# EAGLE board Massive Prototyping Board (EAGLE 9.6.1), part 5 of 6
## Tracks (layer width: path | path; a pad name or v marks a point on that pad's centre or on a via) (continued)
N$1626  (via drill 0.94)
  Bottom 2.032: v262.89,220.98 v265.43,220.98 v267.97,220.98 v270.51,220.98 v273.05,220.98
N$1627  (via drill 0.94)
  Bottom 2.032: v262.89,223.52 v265.43,223.52 v267.97,223.52 v270.51,223.52 v273.05,223.52
N$1628  (via drill 0.94)
  Bottom 2.032: v262.89,226.06 v265.43,226.06 v267.97,226.06 v270.51,226.06 v273.05,226.06
N$1629  (via drill 0.94)
  Bottom 2.032: v262.89,228.6 v265.43,228.6 v267.97,228.6 v270.51,228.6 v273.05,228.6
N$1630  (via drill 0.94)
  Bottom 2.032: v262.89,231.14 v265.43,231.14 v267.97,231.14 v270.51,231.14 v273.05,231.14
N$1631  (via drill 0.94)
  Bottom 2.032: v262.89,233.68 v265.43,233.68 v267.97,233.68 v270.51,233.68 v273.05,233.68
N$1632  (via drill 0.94)
  Bottom 2.032: v262.89,236.22 v265.43,236.22 v267.97,236.22 v270.51,236.22 v273.05,236.22
N$1633  (via drill 0.94)
  Bottom 2.032: v262.89,238.76 v265.43,238.76 v267.97,238.76 v270.51,238.76 v273.05,238.76
N$1634  (via drill 0.94)
  Bottom 2.032: v262.89,241.3 v265.43,241.3 v267.97,241.3 v270.51,241.3 v273.05,241.3
N$1635  (via drill 0.94)
  Bottom 2.032: v262.89,243.84 v265.43,243.84 v267.97,243.84 v270.51,243.84 v273.05,243.84
N$1636  (via drill 0.94)
  Bottom 2.032: v262.89,246.38 v265.43,246.38 v267.97,246.38 v270.51,246.38 v273.05,246.38
N$1637  (via drill 0.94)
  Bottom 2.032: v262.89,248.92 v265.43,248.92 v267.97,248.92 v270.51,248.92 v273.05,248.92
N$1638  (via drill 0.94)
  Bottom 2.032: v262.89,251.46 v265.43,251.46 v267.97,251.46 v270.51,251.46 v273.05,251.46
N$1639  (via drill 0.94)
  Bottom 2.032: v262.89,254 v265.43,254 v267.97,254 v270.51,254 v273.05,254
N$1640  (via drill 0.94)
  Bottom 2.032: v262.89,256.54 v265.43,256.54 v267.97,256.54 v270.51,256.54 v273.05,256.54
N$1641  (via drill 0.94)
  Bottom 2.032: v262.89,259.08 v265.43,259.08 v267.97,259.08 v270.51,259.08 v273.05,259.08
N$1642  (via drill 0.94)
  Bottom 2.032: v262.89,261.62 v265.43,261.62 v267.97,261.62 v270.51,261.62 v273.05,261.62
N$1643  (via drill 0.94)
  Bottom 2.032: v262.89,264.16 v265.43,264.16 v267.97,264.16 v270.51,264.16 v273.05,264.16
N$1644  (via drill 0.94)
  Bottom 2.032: v262.89,266.7 v265.43,266.7 v267.97,266.7 v270.51,266.7 v273.05,266.7
N$1645  (via drill 0.94)
  Bottom 2.032: v262.89,269.24 v265.43,269.24 v267.97,269.24 v270.51,269.24 v273.05,269.24
N$1646  (via drill 0.94)
  Bottom 2.032: v262.89,271.78 v265.43,271.78 v267.97,271.78 v270.51,271.78 v273.05,271.78
N$1647  (via drill 0.94)
  Bottom 2.032: v262.89,274.32 v265.43,274.32 v267.97,274.32 v270.51,274.32 v273.05,274.32
N$1648  (via drill 0.94)
  Bottom 2.032: v262.89,276.86 v265.43,276.86 v267.97,276.86 v270.51,276.86 v273.05,276.86
N$1649  (via drill 0.94)
  Bottom 2.032: v280.67,12.7 v283.21,12.7 v285.75,12.7 v288.29,12.7 v290.83,12.7
N$1650  (via drill 0.94)
  Bottom 2.032: v280.67,15.24 v283.21,15.24 v285.75,15.24 v288.29,15.24 v290.83,15.24
N$1651  (via drill 0.94)
  Bottom 2.032: v280.67,17.78 v283.21,17.78 v285.75,17.78 v288.29,17.78 v290.83,17.78
N$1652  (via drill 0.94)
  Bottom 2.032: v280.67,20.32 v283.21,20.32 v285.75,20.32 v288.29,20.32 v290.83,20.32
N$1653  (via drill 0.94)
  Bottom 2.032: v280.67,22.86 v283.21,22.86 v285.75,22.86 v288.29,22.86 v290.83,22.86
N$1654  (via drill 0.94)
  Bottom 2.032: v280.67,25.4 v283.21,25.4 v285.75,25.4 v288.29,25.4 v290.83,25.4
N$1655  (via drill 0.94)
  Bottom 2.032: v280.67,27.94 v283.21,27.94 v285.75,27.94 v288.29,27.94 v290.83,27.94
N$1656  (via drill 0.94)
  Bottom 2.032: v280.67,30.48 v283.21,30.48 v285.75,30.48 v288.29,30.48 v290.83,30.48
N$1657  (via drill 0.94)
  Bottom 2.032: v280.67,33.02 v283.21,33.02 v285.75,33.02 v288.29,33.02 v290.83,33.02
N$1658  (via drill 0.94)
  Bottom 2.032: v280.67,35.56 v283.21,35.56 v285.75,35.56 v288.29,35.56 v290.83,35.56
N$1659  (via drill 0.94)
  Bottom 2.032: v280.67,38.1 v283.21,38.1 v285.75,38.1 v288.29,38.1 v290.83,38.1
N$1660  (via drill 0.94)
  Bottom 2.032: v280.67,40.64 v283.21,40.64 v285.75,40.64 v288.29,40.64 v290.83,40.64
N$1661  (via drill 0.94)
  Bottom 2.032: v280.67,43.18 v283.21,43.18 v285.75,43.18 v288.29,43.18 v290.83,43.18
N$1662  (via drill 0.94)
  Bottom 2.032: v280.67,45.72 v283.21,45.72 v285.75,45.72 v288.29,45.72 v290.83,45.72
N$1663  (via drill 0.94)
  Bottom 2.032: v280.67,48.26 v283.21,48.26 v285.75,48.26 v288.29,48.26 v290.83,48.26
N$1664  (via drill 0.94)
  Bottom 2.032: v280.67,50.8 v283.21,50.8 v285.75,50.8 v288.29,50.8 v290.83,50.8
N$1665  (via drill 0.94)
  Bottom 2.032: v280.67,53.34 v283.21,53.34 v285.75,53.34 v288.29,53.34 v290.83,53.34
N$1666  (via drill 0.94)
  Bottom 2.032: v280.67,55.88 v283.21,55.88 v285.75,55.88 v288.29,55.88 v290.83,55.88
N$1667  (via drill 0.94)
  Bottom 2.032: v280.67,58.42 v283.21,58.42 v285.75,58.42 v288.29,58.42 v290.83,58.42
N$1668  (via drill 0.94)
  Bottom 2.032: v280.67,60.96 v283.21,60.96 v285.75,60.96 v288.29,60.96 v290.83,60.96
N$1669  (via drill 0.94)
  Bottom 2.032: v280.67,63.5 v283.21,63.5 v285.75,63.5 v288.29,63.5 v290.83,63.5
N$1670  (via drill 0.94)
  Bottom 2.032: v280.67,66.04 v283.21,66.04 v285.75,66.04 v288.29,66.04 v290.83,66.04
N$1671  (via drill 0.94)
  Bottom 2.032: v280.67,68.58 v283.21,68.58 v285.75,68.58 v288.29,68.58 v290.83,68.58
N$1672  (via drill 0.94)
  Bottom 2.032: v280.67,71.12 v283.21,71.12 v285.75,71.12 v288.29,71.12 v290.83,71.12
N$1673  (via drill 0.94)
  Bottom 2.032: v280.67,73.66 v283.21,73.66 v285.75,73.66 v288.29,73.66 v290.83,73.66
N$1674  (via drill 0.94)
  Bottom 2.032: v280.67,76.2 v283.21,76.2 v285.75,76.2 v288.29,76.2 v290.83,76.2
N$1675  (via drill 0.94)
  Bottom 2.032: v280.67,78.74 v283.21,78.74 v285.75,78.74 v288.29,78.74 v290.83,78.74
N$1676  (via drill 0.94)
  Bottom 2.032: v280.67,81.28 v283.21,81.28 v285.75,81.28 v288.29,81.28 v290.83,81.28
N$1677  (via drill 0.94)
  Bottom 2.032: v280.67,83.82 v283.21,83.82 v285.75,83.82 v288.29,83.82 v290.83,83.82
N$1678  (via drill 0.94)
  Bottom 2.032: v280.67,86.36 v283.21,86.36 v285.75,86.36 v288.29,86.36 v290.83,86.36
N$1679  (via drill 0.94)
  Bottom 2.032: v280.67,88.9 v283.21,88.9 v285.75,88.9 v288.29,88.9 v290.83,88.9
N$1680  (via drill 0.94)
  Bottom 2.032: v280.67,91.44 v283.21,91.44 v285.75,91.44 v288.29,91.44 v290.83,91.44
N$1681  (via drill 0.94)
  Bottom 2.032: v280.67,93.98 v283.21,93.98 v285.75,93.98 v288.29,93.98 v290.83,93.98
N$1682  (via drill 0.94)
  Bottom 2.032: v280.67,96.52 v283.21,96.52 v285.75,96.52 v288.29,96.52 v290.83,96.52
N$1683  (via drill 0.94)
  Bottom 2.032: v280.67,99.06 v283.21,99.06 v285.75,99.06 v288.29,99.06 v290.83,99.06
N$1684  (via drill 0.94)
  Bottom 2.032: v280.67,101.6 v283.21,101.6 v285.75,101.6 v288.29,101.6 v290.83,101.6
N$1685  (via drill 0.94)
  Bottom 2.032: v280.67,104.14 v283.21,104.14 v285.75,104.14 v288.29,104.14 v290.83,104.14
N$1686  (via drill 0.94)
  Bottom 2.032: v280.67,106.68 v283.21,106.68 v285.75,106.68 v288.29,106.68 v290.83,106.68
N$1687  (via drill 0.94)
  Bottom 2.032: v280.67,109.22 v283.21,109.22 v285.75,109.22 v288.29,109.22 v290.83,109.22
N$1688  (via drill 0.94)
  Bottom 2.032: v280.67,111.76 v283.21,111.76 v285.75,111.76 v288.29,111.76 v290.83,111.76
N$1689  (via drill 0.94)
  Bottom 2.032: v280.67,114.3 v283.21,114.3 v285.75,114.3 v288.29,114.3 v290.83,114.3
N$1690  (via drill 0.94)
  Bottom 2.032: v280.67,116.84 v283.21,116.84 v285.75,116.84 v288.29,116.84 v290.83,116.84
N$1691  (via drill 0.94)
  Bottom 2.032: v280.67,119.38 v283.21,119.38 v285.75,119.38 v288.29,119.38 v290.83,119.38
N$1692  (via drill 0.94)
  Bottom 2.032: v280.67,121.92 v283.21,121.92 v285.75,121.92 v288.29,121.92 v290.83,121.92
N$1693  (via drill 0.94)
  Bottom 2.032: v280.67,124.46 v283.21,124.46 v285.75,124.46 v288.29,124.46 v290.83,124.46
N$1694  (via drill 0.94)
  Bottom 2.032: v280.67,127 v283.21,127 v285.75,127 v288.29,127 v290.83,127
N$1695  (via drill 0.94)
  Bottom 2.032: v280.67,129.54 v283.21,129.54 v285.75,129.54 v288.29,129.54 v290.83,129.54
N$1696  (via drill 0.94)
  Bottom 2.032: v280.67,132.08 v283.21,132.08 v285.75,132.08 v288.29,132.08 v290.83,132.08
N$1697  (via drill 0.94)
  Bottom 2.032: v280.67,134.62 v283.21,134.62 v285.75,134.62 v288.29,134.62 v290.83,134.62
N$1698  (via drill 0.94)
  Bottom 2.032: v280.67,137.16 v283.21,137.16 v285.75,137.16 v288.29,137.16 v290.83,137.16
N$1699  (via drill 0.94)
  Bottom 2.032: v280.67,139.7 v283.21,139.7 v285.75,139.7 v288.29,139.7 v290.83,139.7
N$1700  (via drill 0.94)
  Bottom 2.032: v280.67,142.24 v283.21,142.24 v285.75,142.24 v288.29,142.24 v290.83,142.24
N$1701  (via drill 0.94)
  Bottom 2.032: v280.67,144.78 v283.21,144.78 v285.75,144.78 v288.29,144.78 v290.83,144.78
N$1702  (via drill 0.94)
  Bottom 2.032: v280.67,147.32 v283.21,147.32 v285.75,147.32 v288.29,147.32 v290.83,147.32
N$1703  (via drill 0.94)
  Bottom 2.032: v280.67,149.86 v283.21,149.86 v285.75,149.86 v288.29,149.86 v290.83,149.86
N$1704  (via drill 0.94)
  Bottom 2.032: v280.67,152.4 v283.21,152.4 v285.75,152.4 v288.29,152.4 v290.83,152.4
N$1705  (via drill 0.94)
  Bottom 2.032: v280.67,154.94 v283.21,154.94 v285.75,154.94 v288.29,154.94 v290.83,154.94
N$1706  (via drill 0.94)
  Bottom 2.032: v280.67,157.48 v283.21,157.48 v285.75,157.48 v288.29,157.48 v290.83,157.48
N$1707  (via drill 0.94)
  Bottom 2.032: v280.67,160.02 v283.21,160.02 v285.75,160.02 v288.29,160.02 v290.83,160.02
N$1708  (via drill 0.94)
  Bottom 2.032: v280.67,162.56 v283.21,162.56 v285.75,162.56 v288.29,162.56 v290.83,162.56
N$1709  (via drill 0.94)
  Bottom 2.032: v280.67,165.1 v283.21,165.1 v285.75,165.1 v288.29,165.1 v290.83,165.1
N$1710  (via drill 0.94)
  Bottom 2.032: v280.67,167.64 v283.21,167.64 v285.75,167.64 v288.29,167.64 v290.83,167.64
N$1711  (via drill 0.94)
  Bottom 2.032: v280.67,170.18 v283.21,170.18 v285.75,170.18 v288.29,170.18 v290.83,170.18
N$1712  (via drill 0.94)
  Bottom 2.032: v280.67,172.72 v283.21,172.72 v285.75,172.72 v288.29,172.72 v290.83,172.72
N$1713  (via drill 0.94)
  Bottom 2.032: v280.67,175.26 v283.21,175.26 v285.75,175.26 v288.29,175.26 v290.83,175.26
N$1714  (via drill 0.94)
  Bottom 2.032: v280.67,177.8 v283.21,177.8 v285.75,177.8 v288.29,177.8 v290.83,177.8
N$1715  (via drill 0.94)
  Bottom 2.032: v280.67,180.34 v283.21,180.34 v285.75,180.34 v288.29,180.34 v290.83,180.34
N$1716  (via drill 0.94)
  Bottom 2.032: v280.67,182.88 v283.21,182.88 v285.75,182.88 v288.29,182.88 v290.83,182.88
N$1717  (via drill 0.94)
  Bottom 2.032: v280.67,185.42 v283.21,185.42 v285.75,185.42 v288.29,185.42 v290.83,185.42
N$1718  (via drill 0.94)
  Bottom 2.032: v280.67,187.96 v283.21,187.96 v285.75,187.96 v288.29,187.96 v290.83,187.96
N$1719  (via drill 0.94)
  Bottom 2.032: v280.67,190.5 v283.21,190.5 v285.75,190.5 v288.29,190.5 v290.83,190.5
N$1720  (via drill 0.94)
  Bottom 2.032: v280.67,193.04 v283.21,193.04 v285.75,193.04 v288.29,193.04 v290.83,193.04
N$1721  (via drill 0.94)
  Bottom 2.032: v280.67,195.58 v283.21,195.58 v285.75,195.58 v288.29,195.58 v290.83,195.58
N$1722  (via drill 0.94)
  Bottom 2.032: v280.67,198.12 v283.21,198.12 v285.75,198.12 v288.29,198.12 v290.83,198.12
N$1723  (via drill 0.94)
  Bottom 2.032: v280.67,200.66 v283.21,200.66 v285.75,200.66 v288.29,200.66 v290.83,200.66
N$1724  (via drill 0.94)
  Bottom 2.032: v280.67,203.2 v283.21,203.2 v285.75,203.2 v288.29,203.2 v290.83,203.2
N$1725  (via drill 0.94)
  Bottom 2.032: v280.67,205.74 v283.21,205.74 v285.75,205.74 v288.29,205.74 v290.83,205.74
N$1726  (via drill 0.94)
  Bottom 2.032: v280.67,208.28 v283.21,208.28 v285.75,208.28 v288.29,208.28 v290.83,208.28
N$1727  (via drill 0.94)
  Bottom 2.032: v280.67,210.82 v283.21,210.82 v285.75,210.82 v288.29,210.82 v290.83,210.82
N$1728  (via drill 0.94)
  Bottom 2.032: v280.67,213.36 v283.21,213.36 v285.75,213.36 v288.29,213.36 v290.83,213.36
N$1729  (via drill 0.94)
  Bottom 2.032: v280.67,215.9 v283.21,215.9 v285.75,215.9 v288.29,215.9 v290.83,215.9
N$1730  (via drill 0.94)
  Bottom 2.032: v280.67,218.44 v283.21,218.44 v285.75,218.44 v288.29,218.44 v290.83,218.44
N$1731  (via drill 0.94)
  Bottom 2.032: v280.67,220.98 v283.21,220.98 v285.75,220.98 v288.29,220.98 v290.83,220.98
N$1732  (via drill 0.94)
  Bottom 2.032: v280.67,223.52 v283.21,223.52 v285.75,223.52 v288.29,223.52 v290.83,223.52
N$1733  (via drill 0.94)
  Bottom 2.032: v280.67,226.06 v283.21,226.06 v285.75,226.06 v288.29,226.06 v290.83,226.06
N$1734  (via drill 0.94)
  Bottom 2.032: v280.67,228.6 v283.21,228.6 v285.75,228.6 v288.29,228.6 v290.83,228.6
N$1735  (via drill 0.94)
  Bottom 2.032: v280.67,231.14 v283.21,231.14 v285.75,231.14 v288.29,231.14 v290.83,231.14
N$1736  (via drill 0.94)
  Bottom 2.032: v280.67,233.68 v283.21,233.68 v285.75,233.68 v288.29,233.68 v290.83,233.68
N$1737  (via drill 0.94)
  Bottom 2.032: v280.67,236.22 v283.21,236.22 v285.75,236.22 v288.29,236.22 v290.83,236.22
N$1738  (via drill 0.94)
  Bottom 2.032: v280.67,238.76 v283.21,238.76 v285.75,238.76 v288.29,238.76 v290.83,238.76
N$1739  (via drill 0.94)
  Bottom 2.032: v280.67,241.3 v283.21,241.3 v285.75,241.3 v288.29,241.3 v290.83,241.3
N$1740  (via drill 0.94)
  Bottom 2.032: v280.67,243.84 v283.21,243.84 v285.75,243.84 v288.29,243.84 v290.83,243.84
N$1741  (via drill 0.94)
  Bottom 2.032: v280.67,246.38 v283.21,246.38 v285.75,246.38 v288.29,246.38 v290.83,246.38
N$1742  (via drill 0.94)
  Bottom 2.032: v280.67,248.92 v283.21,248.92 v285.75,248.92 v288.29,248.92 v290.83,248.92
N$1743  (via drill 0.94)
  Bottom 2.032: v280.67,251.46 v283.21,251.46 v285.75,251.46 v288.29,251.46 v290.83,251.46
N$1744  (via drill 0.94)
  Bottom 2.032: v280.67,254 v283.21,254 v285.75,254 v288.29,254 v290.83,254
N$1745  (via drill 0.94)
  Bottom 2.032: v280.67,256.54 v283.21,256.54 v285.75,256.54 v288.29,256.54 v290.83,256.54
N$1746  (via drill 0.94)
  Bottom 2.032: v280.67,259.08 v283.21,259.08 v285.75,259.08 v288.29,259.08 v290.83,259.08
N$1747  (via drill 0.94)
  Bottom 2.032: v280.67,261.62 v283.21,261.62 v285.75,261.62 v288.29,261.62 v290.83,261.62
N$1748  (via drill 0.94)
  Bottom 2.032: v280.67,264.16 v283.21,264.16 v285.75,264.16 v288.29,264.16 v290.83,264.16
N$1749  (via drill 0.94)
  Bottom 2.032: v280.67,266.7 v283.21,266.7 v285.75,266.7 v288.29,266.7 v290.83,266.7
N$1750  (via drill 0.94)
  Bottom 2.032: v280.67,269.24 v283.21,269.24 v285.75,269.24 v288.29,269.24 v290.83,269.24
N$1751  (via drill 0.94)
  Bottom 2.032: v280.67,271.78 v283.21,271.78 v285.75,271.78 v288.29,271.78 v290.83,271.78
N$1752  (via drill 0.94)
  Bottom 2.032: v280.67,274.32 v283.21,274.32 v285.75,274.32 v288.29,274.32 v290.83,274.32
N$1753  (via drill 0.94)
  Bottom 2.032: v280.67,276.86 v283.21,276.86 v285.75,276.86 v288.29,276.86 v290.83,276.86
N$1754  (via drill 0.94)
  Bottom 2.032: v293.37,12.7 v295.91,12.7 v298.45,12.7 v300.99,12.7 v303.53,12.7
N$1755  (via drill 0.94)
  Bottom 2.032: v293.37,15.24 v295.91,15.24 v298.45,15.24 v300.99,15.24 v303.53,15.24
N$1756  (via drill 0.94)
  Bottom 2.032: v293.37,17.78 v295.91,17.78 v298.45,17.78 v300.99,17.78 v303.53,17.78
N$1757  (via drill 0.94)
  Bottom 2.032: v293.37,20.32 v295.91,20.32 v298.45,20.32 v300.99,20.32 v303.53,20.32
N$1758  (via drill 0.94)
  Bottom 2.032: v293.37,22.86 v295.91,22.86 v298.45,22.86 v300.99,22.86 v303.53,22.86
N$1759  (via drill 0.94)
  Bottom 2.032: v293.37,25.4 v295.91,25.4 v298.45,25.4 v300.99,25.4 v303.53,25.4
N$1760  (via drill 0.94)
  Bottom 2.032: v293.37,27.94 v295.91,27.94 v298.45,27.94 v300.99,27.94 v303.53,27.94
N$1761  (via drill 0.94)
  Bottom 2.032: v293.37,30.48 v295.91,30.48 v298.45,30.48 v300.99,30.48 v303.53,30.48
N$1762  (via drill 0.94)
  Bottom 2.032: v293.37,33.02 v295.91,33.02 v298.45,33.02 v300.99,33.02 v303.53,33.02
N$1763  (via drill 0.94)
  Bottom 2.032: v293.37,35.56 v295.91,35.56 v298.45,35.56 v300.99,35.56 v303.53,35.56
N$1764  (via drill 0.94)
  Bottom 2.032: v293.37,38.1 v295.91,38.1 v298.45,38.1 v300.99,38.1 v303.53,38.1
N$1765  (via drill 0.94)
  Bottom 2.032: v293.37,40.64 v295.91,40.64 v298.45,40.64 v300.99,40.64 v303.53,40.64
N$1766  (via drill 0.94)
  Bottom 2.032: v293.37,43.18 v295.91,43.18 v298.45,43.18 v300.99,43.18 v303.53,43.18
N$1767  (via drill 0.94)
  Bottom 2.032: v293.37,45.72 v295.91,45.72 v298.45,45.72 v300.99,45.72 v303.53,45.72
N$1768  (via drill 0.94)
  Bottom 2.032: v293.37,48.26 v295.91,48.26 v298.45,48.26 v300.99,48.26 v303.53,48.26
N$1769  (via drill 0.94)
  Bottom 2.032: v293.37,50.8 v295.91,50.8 v298.45,50.8 v300.99,50.8 v303.53,50.8
N$1770  (via drill 0.94)
  Bottom 2.032: v293.37,53.34 v295.91,53.34 v298.45,53.34 v300.99,53.34 v303.53,53.34
N$1771  (via drill 0.94)
  Bottom 2.032: v293.37,55.88 v295.91,55.88 v298.45,55.88 v300.99,55.88 v303.53,55.88
N$1772  (via drill 0.94)
  Bottom 2.032: v293.37,58.42 v295.91,58.42 v298.45,58.42 v300.99,58.42 v303.53,58.42
N$1773  (via drill 0.94)
  Bottom 2.032: v293.37,60.96 v295.91,60.96 v298.45,60.96 v300.99,60.96 v303.53,60.96
N$1774  (via drill 0.94)
  Bottom 2.032: v293.37,63.5 v295.91,63.5 v298.45,63.5 v300.99,63.5 v303.53,63.5
N$1775  (via drill 0.94)
  Bottom 2.032: v293.37,66.04 v295.91,66.04 v298.45,66.04 v300.99,66.04 v303.53,66.04
N$1776  (via drill 0.94)
  Bottom 2.032: v293.37,68.58 v295.91,68.58 v298.45,68.58 v300.99,68.58 v303.53,68.58
N$1777  (via drill 0.94)
  Bottom 2.032: v293.37,71.12 v295.91,71.12 v298.45,71.12 v300.99,71.12 v303.53,71.12
N$1778  (via drill 0.94)
  Bottom 2.032: v293.37,73.66 v295.91,73.66 v298.45,73.66 v300.99,73.66 v303.53,73.66
N$1779  (via drill 0.94)
  Bottom 2.032: v293.37,76.2 v295.91,76.2 v298.45,76.2 v300.99,76.2 v303.53,76.2
N$1780  (via drill 0.94)
  Bottom 2.032: v293.37,78.74 v295.91,78.74 v298.45,78.74 v300.99,78.74 v303.53,78.74
N$1781  (via drill 0.94)
  Bottom 2.032: v293.37,81.28 v295.91,81.28 v298.45,81.28 v300.99,81.28 v303.53,81.28
N$1782  (via drill 0.94)
  Bottom 2.032: v293.37,83.82 v295.91,83.82 v298.45,83.82 v300.99,83.82 v303.53,83.82
N$1783  (via drill 0.94)
  Bottom 2.032: v293.37,86.36 v295.91,86.36 v298.45,86.36 v300.99,86.36 v303.53,86.36
N$1784  (via drill 0.94)
  Bottom 2.032: v293.37,88.9 v295.91,88.9 v298.45,88.9 v300.99,88.9 v303.53,88.9
N$1785  (via drill 0.94)
  Bottom 2.032: v293.37,91.44 v295.91,91.44 v298.45,91.44 v300.99,91.44 v303.53,91.44
N$1786  (via drill 0.94)
  Bottom 2.032: v293.37,93.98 v295.91,93.98 v298.45,93.98 v300.99,93.98 v303.53,93.98
N$1787  (via drill 0.94)
  Bottom 2.032: v293.37,96.52 v295.91,96.52 v298.45,96.52 v300.99,96.52 v303.53,96.52
N$1788  (via drill 0.94)
  Bottom 2.032: v293.37,99.06 v295.91,99.06 v298.45,99.06 v300.99,99.06 v303.53,99.06
N$1789  (via drill 0.94)
  Bottom 2.032: v293.37,101.6 v295.91,101.6 v298.45,101.6 v300.99,101.6 v303.53,101.6
N$1790  (via drill 0.94)
  Bottom 2.032: v293.37,104.14 v295.91,104.14 v298.45,104.14 v300.99,104.14 v303.53,104.14
N$1791  (via drill 0.94)
  Bottom 2.032: v293.37,106.68 v295.91,106.68 v298.45,106.68 v300.99,106.68 v303.53,106.68
N$1792  (via drill 0.94)
  Bottom 2.032: v293.37,109.22 v295.91,109.22 v298.45,109.22 v300.99,109.22 v303.53,109.22
N$1793  (via drill 0.94)
  Bottom 2.032: v293.37,111.76 v295.91,111.76 v298.45,111.76 v300.99,111.76 v303.53,111.76
N$1794  (via drill 0.94)
  Bottom 2.032: v293.37,114.3 v295.91,114.3 v298.45,114.3 v300.99,114.3 v303.53,114.3
N$1795  (via drill 0.94)
  Bottom 2.032: v293.37,116.84 v295.91,116.84 v298.45,116.84 v300.99,116.84 v303.53,116.84
N$1796  (via drill 0.94)
  Bottom 2.032: v293.37,119.38 v295.91,119.38 v298.45,119.38 v300.99,119.38 v303.53,119.38
N$1797  (via drill 0.94)
  Bottom 2.032: v293.37,121.92 v295.91,121.92 v298.45,121.92 v300.99,121.92 v303.53,121.92
N$1798  (via drill 0.94)
  Bottom 2.032: v293.37,124.46 v295.91,124.46 v298.45,124.46 v300.99,124.46 v303.53,124.46
N$1799  (via drill 0.94)
  Bottom 2.032: v293.37,127 v295.91,127 v298.45,127 v300.99,127 v303.53,127
N$1800  (via drill 0.94)
  Bottom 2.032: v293.37,129.54 v295.91,129.54 v298.45,129.54 v300.99,129.54 v303.53,129.54
N$1801  (via drill 0.94)
  Bottom 2.032: v293.37,132.08 v295.91,132.08 v298.45,132.08 v300.99,132.08 v303.53,132.08
N$1802  (via drill 0.94)
  Bottom 2.032: v293.37,134.62 v295.91,134.62 v298.45,134.62 v300.99,134.62 v303.53,134.62
N$1803  (via drill 0.94)
  Bottom 2.032: v293.37,137.16 v295.91,137.16 v298.45,137.16 v300.99,137.16 v303.53,137.16
N$1804  (via drill 0.94)
  Bottom 2.032: v293.37,139.7 v295.91,139.7 v298.45,139.7 v300.99,139.7 v303.53,139.7
N$1805  (via drill 0.94)
  Bottom 2.032: v293.37,142.24 v295.91,142.24 v298.45,142.24 v300.99,142.24 v303.53,142.24
N$1806  (via drill 0.94)
  Bottom 2.032: v293.37,144.78 v295.91,144.78 v298.45,144.78 v300.99,144.78 v303.53,144.78
N$1807  (via drill 0.94)
  Bottom 2.032: v293.37,147.32 v295.91,147.32 v298.45,147.32 v300.99,147.32 v303.53,147.32
N$1808  (via drill 0.94)
  Bottom 2.032: v293.37,149.86 v295.91,149.86 v298.45,149.86 v300.99,149.86 v303.53,149.86
N$1809  (via drill 0.94)
  Bottom 2.032: v293.37,152.4 v295.91,152.4 v298.45,152.4 v300.99,152.4 v303.53,152.4
N$1810  (via drill 0.94)
  Bottom 2.032: v293.37,154.94 v295.91,154.94 v298.45,154.94 v300.99,154.94 v303.53,154.94
N$1811  (via drill 0.94)
  Bottom 2.032: v293.37,157.48 v295.91,157.48 v298.45,157.48 v300.99,157.48 v303.53,157.48
N$1812  (via drill 0.94)
  Bottom 2.032: v293.37,160.02 v295.91,160.02 v298.45,160.02 v300.99,160.02 v303.53,160.02
N$1813  (via drill 0.94)
  Bottom 2.032: v293.37,162.56 v295.91,162.56 v298.45,162.56 v300.99,162.56 v303.53,162.56
N$1814  (via drill 0.94)
  Bottom 2.032: v293.37,165.1 v295.91,165.1 v298.45,165.1 v300.99,165.1 v303.53,165.1
N$1815  (via drill 0.94)
  Bottom 2.032: v293.37,167.64 v295.91,167.64 v298.45,167.64 v300.99,167.64 v303.53,167.64
N$1816  (via drill 0.94)
  Bottom 2.032: v293.37,170.18 v295.91,170.18 v298.45,170.18 v300.99,170.18 v303.53,170.18
N$1817  (via drill 0.94)
  Bottom 2.032: v293.37,172.72 v295.91,172.72 v298.45,172.72 v300.99,172.72 v303.53,172.72
N$1818  (via drill 0.94)
  Bottom 2.032: v293.37,175.26 v295.91,175.26 v298.45,175.26 v300.99,175.26 v303.53,175.26
N$1819  (via drill 0.94)
  Bottom 2.032: v293.37,177.8 v295.91,177.8 v298.45,177.8 v300.99,177.8 v303.53,177.8
N$1820  (via drill 0.94)
  Bottom 2.032: v293.37,180.34 v295.91,180.34 v298.45,180.34 v300.99,180.34 v303.53,180.34
N$1821  (via drill 0.94)
  Bottom 2.032: v293.37,182.88 v295.91,182.88 v298.45,182.88 v300.99,182.88 v303.53,182.88
N$1822  (via drill 0.94)
  Bottom 2.032: v293.37,185.42 v295.91,185.42 v298.45,185.42 v300.99,185.42 v303.53,185.42
N$1823  (via drill 0.94)
  Bottom 2.032: v293.37,187.96 v295.91,187.96 v298.45,187.96 v300.99,187.96 v303.53,187.96
N$1824  (via drill 0.94)
  Bottom 2.032: v293.37,190.5 v295.91,190.5 v298.45,190.5 v300.99,190.5 v303.53,190.5
N$1825  (via drill 0.94)
  Bottom 2.032: v293.37,193.04 v295.91,193.04 v298.45,193.04 v300.99,193.04 v303.53,193.04
N$1826  (via drill 0.94)
  Bottom 2.032: v293.37,195.58 v295.91,195.58 v298.45,195.58 v300.99,195.58 v303.53,195.58
N$1827  (via drill 0.94)
  Bottom 2.032: v293.37,198.12 v295.91,198.12 v298.45,198.12 v300.99,198.12 v303.53,198.12
N$1828  (via drill 0.94)
  Bottom 2.032: v293.37,200.66 v295.91,200.66 v298.45,200.66 v300.99,200.66 v303.53,200.66
N$1829  (via drill 0.94)
  Bottom 2.032: v293.37,203.2 v295.91,203.2 v298.45,203.2 v300.99,203.2 v303.53,203.2
N$1830  (via drill 0.94)
  Bottom 2.032: v293.37,205.74 v295.91,205.74 v298.45,205.74 v300.99,205.74 v303.53,205.74
N$1831  (via drill 0.94)
  Bottom 2.032: v293.37,208.28 v295.91,208.28 v298.45,208.28 v300.99,208.28 v303.53,208.28
N$1832  (via drill 0.94)
  Bottom 2.032: v293.37,210.82 v295.91,210.82 v298.45,210.82 v300.99,210.82 v303.53,210.82
N$1833  (via drill 0.94)
  Bottom 2.032: v293.37,213.36 v295.91,213.36 v298.45,213.36 v300.99,213.36 v303.53,213.36
N$1834  (via drill 0.94)
  Bottom 2.032: v293.37,215.9 v295.91,215.9 v298.45,215.9 v300.99,215.9 v303.53,215.9
N$1835  (via drill 0.94)
  Bottom 2.032: v293.37,218.44 v295.91,218.44 v298.45,218.44 v300.99,218.44 v303.53,218.44
N$1836  (via drill 0.94)
  Bottom 2.032: v293.37,220.98 v295.91,220.98 v298.45,220.98 v300.99,220.98 v303.53,220.98
N$1837  (via drill 0.94)
  Bottom 2.032: v293.37,223.52 v295.91,223.52 v298.45,223.52 v300.99,223.52 v303.53,223.52
N$1838  (via drill 0.94)
  Bottom 2.032: v293.37,226.06 v295.91,226.06 v298.45,226.06 v300.99,226.06 v303.53,226.06
N$1839  (via drill 0.94)
  Bottom 2.032: v293.37,228.6 v295.91,228.6 v298.45,228.6 v300.99,228.6 v303.53,228.6
N$1840  (via drill 0.94)
  Bottom 2.032: v293.37,231.14 v295.91,231.14 v298.45,231.14 v300.99,231.14 v303.53,231.14
N$1841  (via drill 0.94)
  Bottom 2.032: v293.37,233.68 v295.91,233.68 v298.45,233.68 v300.99,233.68 v303.53,233.68
N$1842  (via drill 0.94)
  Bottom 2.032: v293.37,236.22 v295.91,236.22 v298.45,236.22 v300.99,236.22 v303.53,236.22
N$1843  (via drill 0.94)
  Bottom 2.032: v293.37,238.76 v295.91,238.76 v298.45,238.76 v300.99,238.76 v303.53,238.76
N$1844  (via drill 0.94)
  Bottom 2.032: v293.37,241.3 v295.91,241.3 v298.45,241.3 v300.99,241.3 v303.53,241.3
N$1845  (via drill 0.94)
  Bottom 2.032: v293.37,243.84 v295.91,243.84 v298.45,243.84 v300.99,243.84 v303.53,243.84
N$1846  (via drill 0.94)
  Bottom 2.032: v293.37,246.38 v295.91,246.38 v298.45,246.38 v300.99,246.38 v303.53,246.38
N$1847  (via drill 0.94)
  Bottom 2.032: v293.37,248.92 v295.91,248.92 v298.45,248.92 v300.99,248.92 v303.53,248.92
N$1848  (via drill 0.94)
  Bottom 2.032: v293.37,251.46 v295.91,251.46 v298.45,251.46 v300.99,251.46 v303.53,251.46
N$1849  (via drill 0.94)
  Bottom 2.032: v293.37,254 v295.91,254 v298.45,254 v300.99,254 v303.53,254
N$1850  (via drill 0.94)
  Bottom 2.032: v293.37,256.54 v295.91,256.54 v298.45,256.54 v300.99,256.54 v303.53,256.54
N$1851  (via drill 0.94)
  Bottom 2.032: v293.37,259.08 v295.91,259.08 v298.45,259.08 v300.99,259.08 v303.53,259.08
N$1852  (via drill 0.94)
  Bottom 2.032: v293.37,261.62 v295.91,261.62 v298.45,261.62 v300.99,261.62 v303.53,261.62
N$1853  (via drill 0.94)
  Bottom 2.032: v293.37,264.16 v295.91,264.16 v298.45,264.16 v300.99,264.16 v303.53,264.16
N$1854  (via drill 0.94)
  Bottom 2.032: v293.37,266.7 v295.91,266.7 v298.45,266.7 v300.99,266.7 v303.53,266.7
N$1855  (via drill 0.94)
  Bottom 2.032: v293.37,269.24 v295.91,269.24 v298.45,269.24 v300.99,269.24 v303.53,269.24
N$1856  (via drill 0.94)
  Bottom 2.032: v293.37,271.78 v295.91,271.78 v298.45,271.78 v300.99,271.78 v303.53,271.78
N$1857  (via drill 0.94)
  Bottom 2.032: v293.37,274.32 v295.91,274.32 v298.45,274.32 v300.99,274.32 v303.53,274.32
N$1858  (via drill 0.94)
  Bottom 2.032: v293.37,276.86 v295.91,276.86 v298.45,276.86 v300.99,276.86 v303.53,276.86
N$1859  (via drill 0.94)
  Bottom 2.032: v311.15,12.7 v313.69,12.7 v316.23,12.7 v318.77,12.7 v321.31,12.7
N$1860  (via drill 0.94)
  Bottom 2.032: v311.15,15.24 v313.69,15.24 v316.23,15.24 v318.77,15.24 v321.31,15.24
N$1861  (via drill 0.94)
  Bottom 2.032: v311.15,17.78 v313.69,17.78 v316.23,17.78 v318.77,17.78 v321.31,17.78
N$1862  (via drill 0.94)
  Bottom 2.032: v311.15,20.32 v313.69,20.32 v316.23,20.32 v318.77,20.32 v321.31,20.32
N$1863  (via drill 0.94)
  Bottom 2.032: v311.15,22.86 v313.69,22.86 v316.23,22.86 v318.77,22.86 v321.31,22.86
N$1864  (via drill 0.94)
  Bottom 2.032: v311.15,25.4 v313.69,25.4 v316.23,25.4 v318.77,25.4 v321.31,25.4
N$1865  (via drill 0.94)
  Bottom 2.032: v311.15,27.94 v313.69,27.94 v316.23,27.94 v318.77,27.94 v321.31,27.94
N$1866  (via drill 0.94)
  Bottom 2.032: v311.15,30.48 v313.69,30.48 v316.23,30.48 v318.77,30.48 v321.31,30.48
N$1867  (via drill 0.94)
  Bottom 2.032: v311.15,33.02 v313.69,33.02 v316.23,33.02 v318.77,33.02 v321.31,33.02
N$1868  (via drill 0.94)
  Bottom 2.032: v311.15,35.56 v313.69,35.56 v316.23,35.56 v318.77,35.56 v321.31,35.56
N$1869  (via drill 0.94)
  Bottom 2.032: v311.15,38.1 v313.69,38.1 v316.23,38.1 v318.77,38.1 v321.31,38.1
N$1870  (via drill 0.94)
  Bottom 2.032: v311.15,40.64 v313.69,40.64 v316.23,40.64 v318.77,40.64 v321.31,40.64
N$1871  (via drill 0.94)
  Bottom 2.032: v311.15,43.18 v313.69,43.18 v316.23,43.18 v318.77,43.18 v321.31,43.18
N$1872  (via drill 0.94)
  Bottom 2.032: v311.15,45.72 v313.69,45.72 v316.23,45.72 v318.77,45.72 v321.31,45.72
N$1873  (via drill 0.94)
  Bottom 2.032: v311.15,48.26 v313.69,48.26 v316.23,48.26 v318.77,48.26 v321.31,48.26
N$1874  (via drill 0.94)
  Bottom 2.032: v311.15,50.8 v313.69,50.8 v316.23,50.8 v318.77,50.8 v321.31,50.8
N$1875  (via drill 0.94)
  Bottom 2.032: v311.15,53.34 v313.69,53.34 v316.23,53.34 v318.77,53.34 v321.31,53.34
N$1876  (via drill 0.94)
  Bottom 2.032: v311.15,55.88 v313.69,55.88 v316.23,55.88 v318.77,55.88 v321.31,55.88
N$1877  (via drill 0.94)
  Bottom 2.032: v311.15,58.42 v313.69,58.42 v316.23,58.42 v318.77,58.42 v321.31,58.42
N$1878  (via drill 0.94)
  Bottom 2.032: v311.15,60.96 v313.69,60.96 v316.23,60.96 v318.77,60.96 v321.31,60.96
N$1879  (via drill 0.94)
  Bottom 2.032: v311.15,63.5 v313.69,63.5 v316.23,63.5 v318.77,63.5 v321.31,63.5
N$1880  (via drill 0.94)
  Bottom 2.032: v311.15,66.04 v313.69,66.04 v316.23,66.04 v318.77,66.04 v321.31,66.04
N$1881  (via drill 0.94)
  Bottom 2.032: v311.15,68.58 v313.69,68.58 v316.23,68.58 v318.77,68.58 v321.31,68.58
N$1882  (via drill 0.94)
  Bottom 2.032: v311.15,71.12 v313.69,71.12 v316.23,71.12 v318.77,71.12 v321.31,71.12
N$1883  (via drill 0.94)
  Bottom 2.032: v311.15,73.66 v313.69,73.66 v316.23,73.66 v318.77,73.66 v321.31,73.66
N$1884  (via drill 0.94)
  Bottom 2.032: v311.15,76.2 v313.69,76.2 v316.23,76.2 v318.77,76.2 v321.31,76.2
N$1885  (via drill 0.94)
  Bottom 2.032: v311.15,78.74 v313.69,78.74 v316.23,78.74 v318.77,78.74 v321.31,78.74
N$1886  (via drill 0.94)
  Bottom 2.032: v311.15,81.28 v313.69,81.28 v316.23,81.28 v318.77,81.28 v321.31,81.28
N$1887  (via drill 0.94)
  Bottom 2.032: v311.15,83.82 v313.69,83.82 v316.23,83.82 v318.77,83.82 v321.31,83.82
N$1888  (via drill 0.94)
  Bottom 2.032: v311.15,86.36 v313.69,86.36 v316.23,86.36 v318.77,86.36 v321.31,86.36
N$1889  (via drill 0.94)
  Bottom 2.032: v311.15,88.9 v313.69,88.9 v316.23,88.9 v318.77,88.9 v321.31,88.9
N$1890  (via drill 0.94)
  Bottom 2.032: v311.15,91.44 v313.69,91.44 v316.23,91.44 v318.77,91.44 v321.31,91.44
N$1891  (via drill 0.94)
  Bottom 2.032: v311.15,93.98 v313.69,93.98 v316.23,93.98 v318.77,93.98 v321.31,93.98
N$1892  (via drill 0.94)
  Bottom 2.032: v311.15,96.52 v313.69,96.52 v316.23,96.52 v318.77,96.52 v321.31,96.52
N$1893  (via drill 0.94)
  Bottom 2.032: v311.15,99.06 v313.69,99.06 v316.23,99.06 v318.77,99.06 v321.31,99.06
N$1894  (via drill 0.94)
  Bottom 2.032: v311.15,101.6 v313.69,101.6 v316.23,101.6 v318.77,101.6 v321.31,101.6
N$1895  (via drill 0.94)
  Bottom 2.032: v311.15,104.14 v313.69,104.14 v316.23,104.14 v318.77,104.14 v321.31,104.14
N$1896  (via drill 0.94)
  Bottom 2.032: v311.15,106.68 v313.69,106.68 v316.23,106.68 v318.77,106.68 v321.31,106.68
N$1897  (via drill 0.94)
  Bottom 2.032: v311.15,109.22 v313.69,109.22 v316.23,109.22 v318.77,109.22 v321.31,109.22
N$1898  (via drill 0.94)
  Bottom 2.032: v311.15,111.76 v313.69,111.76 v316.23,111.76 v318.77,111.76 v321.31,111.76
N$1899  (via drill 0.94)
  Bottom 2.032: v311.15,114.3 v313.69,114.3 v316.23,114.3 v318.77,114.3 v321.31,114.3
N$1900  (via drill 0.94)
  Bottom 2.032: v311.15,116.84 v313.69,116.84 v316.23,116.84 v318.77,116.84 v321.31,116.84
N$1901  (via drill 0.94)
  Bottom 2.032: v311.15,119.38 v313.69,119.38 v316.23,119.38 v318.77,119.38 v321.31,119.38
N$1902  (via drill 0.94)
  Bottom 2.032: v311.15,121.92 v313.69,121.92 v316.23,121.92 v318.77,121.92 v321.31,121.92
N$1903  (via drill 0.94)
  Bottom 2.032: v311.15,124.46 v313.69,124.46 v316.23,124.46 v318.77,124.46 v321.31,124.46
N$1904  (via drill 0.94)
  Bottom 2.032: v311.15,127 v313.69,127 v316.23,127 v318.77,127 v321.31,127
N$1905  (via drill 0.94)
  Bottom 2.032: v311.15,129.54 v313.69,129.54 v316.23,129.54 v318.77,129.54 v321.31,129.54
N$1906  (via drill 0.94)
  Bottom 2.032: v311.15,132.08 v313.69,132.08 v316.23,132.08 v318.77,132.08 v321.31,132.08
N$1907  (via drill 0.94)
  Bottom 2.032: v311.15,134.62 v313.69,134.62 v316.23,134.62 v318.77,134.62 v321.31,134.62
N$1908  (via drill 0.94)
  Bottom 2.032: v311.15,137.16 v313.69,137.16 v316.23,137.16 v318.77,137.16 v321.31,137.16
N$1909  (via drill 0.94)
  Bottom 2.032: v311.15,139.7 v313.69,139.7 v316.23,139.7 v318.77,139.7 v321.31,139.7
N$1910  (via drill 0.94)
  Bottom 2.032: v311.15,142.24 v313.69,142.24 v316.23,142.24 v318.77,142.24 v321.31,142.24
N$1911  (via drill 0.94)
  Bottom 2.032: v311.15,144.78 v313.69,144.78 v316.23,144.78 v318.77,144.78 v321.31,144.78
N$1912  (via drill 0.94)
  Bottom 2.032: v311.15,147.32 v313.69,147.32 v316.23,147.32 v318.77,147.32 v321.31,147.32
N$1913  (via drill 0.94)
  Bottom 2.032: v311.15,149.86 v313.69,149.86 v316.23,149.86 v318.77,149.86 v321.31,149.86
N$1914  (via drill 0.94)
  Bottom 2.032: v311.15,152.4 v313.69,152.4 v316.23,152.4 v318.77,152.4 v321.31,152.4
N$1915  (via drill 0.94)
  Bottom 2.032: v311.15,154.94 v313.69,154.94 v316.23,154.94 v318.77,154.94 v321.31,154.94
N$1916  (via drill 0.94)
  Bottom 2.032: v311.15,157.48 v313.69,157.48 v316.23,157.48 v318.77,157.48 v321.31,157.48
N$1917  (via drill 0.94)
  Bottom 2.032: v311.15,160.02 v313.69,160.02 v316.23,160.02 v318.77,160.02 v321.31,160.02
N$1918  (via drill 0.94)
  Bottom 2.032: v311.15,162.56 v313.69,162.56 v316.23,162.56 v318.77,162.56 v321.31,162.56
N$1919  (via drill 0.94)
  Bottom 2.032: v311.15,165.1 v313.69,165.1 v316.23,165.1 v318.77,165.1 v321.31,165.1
N$1920  (via drill 0.94)
  Bottom 2.032: v311.15,167.64 v313.69,167.64 v316.23,167.64 v318.77,167.64 v321.31,167.64
N$1921  (via drill 0.94)
  Bottom 2.032: v311.15,170.18 v313.69,170.18 v316.23,170.18 v318.77,170.18 v321.31,170.18
N$1922  (via drill 0.94)
  Bottom 2.032: v311.15,172.72 v313.69,172.72 v316.23,172.72 v318.77,172.72 v321.31,172.72
N$1923  (via drill 0.94)
  Bottom 2.032: v311.15,175.26 v313.69,175.26 v316.23,175.26 v318.77,175.26 v321.31,175.26
N$1924  (via drill 0.94)
  Bottom 2.032: v311.15,177.8 v313.69,177.8 v316.23,177.8 v318.77,177.8 v321.31,177.8
N$1925  (via drill 0.94)
  Bottom 2.032: v311.15,180.34 v313.69,180.34 v316.23,180.34 v318.77,180.34 v321.31,180.34
N$1926  (via drill 0.94)
  Bottom 2.032: v311.15,182.88 v313.69,182.88 v316.23,182.88 v318.77,182.88 v321.31,182.88
N$1927  (via drill 0.94)
  Bottom 2.032: v311.15,185.42 v313.69,185.42 v316.23,185.42 v318.77,185.42 v321.31,185.42
N$1928  (via drill 0.94)
  Bottom 2.032: v311.15,187.96 v313.69,187.96 v316.23,187.96 v318.77,187.96 v321.31,187.96
N$1929  (via drill 0.94)
  Bottom 2.032: v311.15,190.5 v313.69,190.5 v316.23,190.5 v318.77,190.5 v321.31,190.5
N$1930  (via drill 0.94)
  Bottom 2.032: v311.15,193.04 v313.69,193.04 v316.23,193.04 v318.77,193.04 v321.31,193.04
N$1931  (via drill 0.94)
  Bottom 2.032: v311.15,195.58 v313.69,195.58 v316.23,195.58 v318.77,195.58 v321.31,195.58
N$1932  (via drill 0.94)
  Bottom 2.032: v311.15,198.12 v313.69,198.12 v316.23,198.12 v318.77,198.12 v321.31,198.12
N$1933  (via drill 0.94)
  Bottom 2.032: v311.15,200.66 v313.69,200.66 v316.23,200.66 v318.77,200.66 v321.31,200.66
N$1934  (via drill 0.94)
  Bottom 2.032: v311.15,203.2 v313.69,203.2 v316.23,203.2 v318.77,203.2 v321.31,203.2
N$1935  (via drill 0.94)
  Bottom 2.032: v311.15,205.74 v313.69,205.74 v316.23,205.74 v318.77,205.74 v321.31,205.74
N$1936  (via drill 0.94)
  Bottom 2.032: v311.15,208.28 v313.69,208.28 v316.23,208.28 v318.77,208.28 v321.31,208.28
N$1937  (via drill 0.94)
  Bottom 2.032: v311.15,210.82 v313.69,210.82 v316.23,210.82 v318.77,210.82 v321.31,210.82
N$1938  (via drill 0.94)
  Bottom 2.032: v311.15,213.36 v313.69,213.36 v316.23,213.36 v318.77,213.36 v321.31,213.36
N$1939  (via drill 0.94)
  Bottom 2.032: v311.15,215.9 v313.69,215.9 v316.23,215.9 v318.77,215.9 v321.31,215.9
N$1940  (via drill 0.94)
  Bottom 2.032: v311.15,218.44 v313.69,218.44 v316.23,218.44 v318.77,218.44 v321.31,218.44
N$1941  (via drill 0.94)
  Bottom 2.032: v311.15,220.98 v313.69,220.98 v316.23,220.98 v318.77,220.98 v321.31,220.98
N$1942  (via drill 0.94)
  Bottom 2.032: v311.15,223.52 v313.69,223.52 v316.23,223.52 v318.77,223.52 v321.31,223.52
N$1943  (via drill 0.94)
  Bottom 2.032: v311.15,226.06 v313.69,226.06 v316.23,226.06 v318.77,226.06 v321.31,226.06
N$1944  (via drill 0.94)
  Bottom 2.032: v311.15,228.6 v313.69,228.6 v316.23,228.6 v318.77,228.6 v321.31,228.6
N$1945  (via drill 0.94)
  Bottom 2.032: v311.15,231.14 v313.69,231.14 v316.23,231.14 v318.77,231.14 v321.31,231.14
N$1946  (via drill 0.94)
  Bottom 2.032: v311.15,233.68 v313.69,233.68 v316.23,233.68 v318.77,233.68 v321.31,233.68
N$1947  (via drill 0.94)
  Bottom 2.032: v311.15,236.22 v313.69,236.22 v316.23,236.22 v318.77,236.22 v321.31,236.22
N$1948  (via drill 0.94)
  Bottom 2.032: v311.15,238.76 v313.69,238.76 v316.23,238.76 v318.77,238.76 v321.31,238.76
N$1949  (via drill 0.94)
  Bottom 2.032: v311.15,241.3 v313.69,241.3 v316.23,241.3 v318.77,241.3 v321.31,241.3
N$1950  (via drill 0.94)
  Bottom 2.032: v311.15,243.84 v313.69,243.84 v316.23,243.84 v318.77,243.84 v321.31,243.84
N$1951  (via drill 0.94)
  Bottom 2.032: v311.15,246.38 v313.69,246.38 v316.23,246.38 v318.77,246.38 v321.31,246.38
N$1952  (via drill 0.94)
  Bottom 2.032: v311.15,248.92 v313.69,248.92 v316.23,248.92 v318.77,248.92 v321.31,248.92
N$1953  (via drill 0.94)
  Bottom 2.032: v311.15,251.46 v313.69,251.46 v316.23,251.46 v318.77,251.46 v321.31,251.46
N$1954  (via drill 0.94)
  Bottom 2.032: v311.15,254 v313.69,254 v316.23,254 v318.77,254 v321.31,254
N$1955  (via drill 0.94)
  Bottom 2.032: v311.15,256.54 v313.69,256.54 v316.23,256.54 v318.77,256.54 v321.31,256.54
N$1956  (via drill 0.94)
  Bottom 2.032: v311.15,259.08 v313.69,259.08 v316.23,259.08 v318.77,259.08 v321.31,259.08
N$1957  (via drill 0.94)
  Bottom 2.032: v311.15,261.62 v313.69,261.62 v316.23,261.62 v318.77,261.62 v321.31,261.62
N$1958  (via drill 0.94)
  Bottom 2.032: v311.15,264.16 v313.69,264.16 v316.23,264.16 v318.77,264.16 v321.31,264.16
N$1959  (via drill 0.94)
  Bottom 2.032: v311.15,266.7 v313.69,266.7 v316.23,266.7 v318.77,266.7 v321.31,266.7
N$1960  (via drill 0.94)
  Bottom 2.032: v311.15,269.24 v313.69,269.24 v316.23,269.24 v318.77,269.24 v321.31,269.24
N$1961  (via drill 0.94)
  Bottom 2.032: v311.15,271.78 v313.69,271.78 v316.23,271.78 v318.77,271.78 v321.31,271.78
N$1962  (via drill 0.94)
  Bottom 2.032: v311.15,274.32 v313.69,274.32 v316.23,274.32 v318.77,274.32 v321.31,274.32
N$1963  (via drill 0.94)
  Bottom 2.032: v311.15,276.86 v313.69,276.86 v316.23,276.86 v318.77,276.86 v321.31,276.86
N$1964  (via drill 0.94)
  Bottom 2.032: v49.53,10.16 v52.07,10.16 v54.61,10.16 v57.15,10.16 v59.69,10.16
N$1965  (via drill 0.94)
  Bottom 2.032: v67.31,10.16 v69.85,10.16 v72.39,10.16 v74.93,10.16 v77.47,10.16
N$1966  (via drill 0.94)
  Bottom 2.032: v80.01,10.16 v82.55,10.16 v85.09,10.16 v87.63,10.16 v90.17,10.16
N$1967  (via drill 0.94)
  Bottom 2.032: v97.79,10.16 v100.33,10.16 v102.87,10.16 v105.41,10.16 v107.95,10.16
N$1968  (via drill 0.94)
  Bottom 2.032: v110.49,10.16 v113.03,10.16 v115.57,10.16 v118.11,10.16 v120.65,10.16
N$1969  (via drill 0.94)
  Bottom 2.032: v128.27,10.16 v130.81,10.16 v133.35,10.16 v135.89,10.16 v138.43,10.16
N$1970  (via drill 0.94)
  Bottom 2.032: v140.97,10.16 v143.51,10.16 v146.05,10.16 v148.59,10.16 v151.13,10.16
N$1971  (via drill 0.94)
  Bottom 2.032: v158.75,10.16 v161.29,10.16 v163.83,10.16 v166.37,10.16 v168.91,10.16
N$1972  (via drill 0.94)
  Bottom 2.032: v171.45,10.16 v173.99,10.16 v176.53,10.16 v179.07,10.16 v181.61,10.16
N$1973  (via drill 0.94)
  Bottom 2.032: v189.23,10.16 v191.77,10.16 v194.31,10.16 v196.85,10.16 v199.39,10.16
N$1974  (via drill 0.94)
  Bottom 2.032: v201.93,10.16 v204.47,10.16 v207.01,10.16 v209.55,10.16 v212.09,10.16
N$1975  (via drill 0.94)
  Bottom 2.032: v219.71,10.16 v222.25,10.16 v224.79,10.16 v227.33,10.16 v229.87,10.16
N$1976  (via drill 0.94)
  Bottom 2.032: v232.41,10.16 v234.95,10.16 v237.49,10.16 v240.03,10.16 v242.57,10.16
N$1977  (via drill 0.94)
  Bottom 2.032: v250.19,10.16 v252.73,10.16 v255.27,10.16 v257.81,10.16 v260.35,10.16
N$1978  (via drill 0.94)
  Bottom 2.032: v262.89,10.16 v265.43,10.16 v267.97,10.16 v270.51,10.16 v273.05,10.16
N$1979  (via drill 0.94)
  Bottom 2.032: v280.67,10.16 v283.21,10.16 v285.75,10.16 v288.29,10.16 v290.83,10.16
N$1980  (via drill 0.94)
  Bottom 2.032: v293.37,10.16 v295.91,10.16 v298.45,10.16 v300.99,10.16 v303.53,10.16
N$1981  (via drill 0.94)
  Bottom 2.032: v311.15,10.16 v313.69,10.16 v316.23,10.16 v318.77,10.16 v321.31,10.16
N$1982  (via drill 0.94)
  Bottom 2.032: v49.53,279.4 v52.07,279.4 v54.61,279.4 v57.15,279.4 v59.69,279.4
N$1983  (via drill 0.94)
  Bottom 2.032: v67.31,279.4 v69.85,279.4 v72.39,279.4 v74.93,279.4 v77.47,279.4
N$1984  (via drill 0.94)
  Bottom 2.032: v80.01,279.4 v82.55,279.4 v85.09,279.4 v87.63,279.4 v90.17,279.4
N$1985  (via drill 0.94)
  Bottom 2.032: v97.79,279.4 v100.33,279.4 v102.87,279.4 v105.41,279.4 v107.95,279.4
N$1986  (via drill 0.94)
  Bottom 2.032: v110.49,279.4 v113.03,279.4 v115.57,279.4 v118.11,279.4 v120.65,279.4
N$1987  (via drill 0.94)
  Bottom 2.032: v128.27,279.4 v130.81,279.4 v133.35,279.4 v135.89,279.4 v138.43,279.4
N$1988  (via drill 0.94)
  Bottom 2.032: v140.97,279.4 v143.51,279.4 v146.05,279.4 v148.59,279.4 v151.13,279.4
N$1989  (via drill 0.94)
  Bottom 2.032: v158.75,279.4 v161.29,279.4 v163.83,279.4 v166.37,279.4 v168.91,279.4
N$1990  (via drill 0.94)
  Bottom 2.032: v171.45,279.4 v173.99,279.4 v176.53,279.4 v179.07,279.4 v181.61,279.4
N$1991  (via drill 0.94)
  Bottom 2.032: v189.23,279.4 v191.77,279.4 v194.31,279.4 v196.85,279.4 v199.39,279.4
N$1992  (via drill 0.94)
  Bottom 2.032: v201.93,279.4 v204.47,279.4 v207.01,279.4 v209.55,279.4 v212.09,279.4
N$1993  (via drill 0.94)
  Bottom 2.032: v219.71,279.4 v222.25,279.4 v224.79,279.4 v227.33,279.4 v229.87,279.4
N$1994  (via drill 0.94)
  Bottom 2.032: v232.41,279.4 v234.95,279.4 v237.49,279.4 v240.03,279.4 v242.57,279.4
N$1995  (via drill 0.94)
  Bottom 2.032: v250.19,279.4 v252.73,279.4 v255.27,279.4 v257.81,279.4 v260.35,279.4
N$1996  (via drill 0.94)
  Bottom 2.032: v262.89,279.4 v265.43,279.4 v267.97,279.4 v270.51,279.4 v273.05,279.4
N$1997  (via drill 0.94)
  Bottom 2.032: v280.67,279.4 v283.21,279.4 v285.75,279.4 v288.29,279.4 v290.83,279.4
N$1998  (via drill 0.94)
  Bottom 2.032: v293.37,279.4 v295.91,279.4 v298.45,279.4 v300.99,279.4 v303.53,279.4
N$1999  (via drill 0.94)
  Bottom 2.032: v311.15,279.4 v313.69,279.4 v316.23,279.4 v318.77,279.4 v321.31,279.4
N$2000  (via drill 0.94)
  Bottom 2.032: v36.83,198.12 v39.37,198.12 v41.91,198.12 v44.45,198.12 v46.99,198.12
N$2001  (via drill 0.94)
  Bottom 2.032: v36.83,200.66 v39.37,200.66 v41.91,200.66 v44.45,200.66 v46.99,200.66
N$2002  (via drill 0.94)
  Bottom 2.032: v36.83,203.2 v39.37,203.2 v41.91,203.2 v44.45,203.2 v46.99,203.2
N$2003  (via drill 0.94)
  Bottom 2.032: v36.83,205.74 v39.37,205.74 v41.91,205.74 v44.45,205.74 v46.99,205.74
N$2004  (via drill 0.94)
  Bottom 2.032: v36.83,208.28 v39.37,208.28 v41.91,208.28 v44.45,208.28 v46.99,208.28
N$2005  (via drill 0.94)
  Bottom 2.032: v36.83,210.82 v39.37,210.82 v41.91,210.82 v44.45,210.82 v46.99,210.82
N$2006  (via drill 0.94)
  Bottom 2.032: v36.83,213.36 v39.37,213.36 v41.91,213.36 v44.45,213.36 v46.99,213.36
N$2007  (via drill 0.94)
  Bottom 2.032: v36.83,215.9 v39.37,215.9 v41.91,215.9 v44.45,215.9 v46.99,215.9
N$2008  (via drill 0.94)
  Bottom 2.032: v36.83,218.44 v39.37,218.44 v41.91,218.44 v44.45,218.44 v46.99,218.44
N$2009  (via drill 0.94)
  Bottom 2.032: v36.83,220.98 v39.37,220.98 v41.91,220.98 v44.45,220.98 v46.99,220.98
N$2010  (via drill 0.94)
  Bottom 2.032: v36.83,223.52 v39.37,223.52 v41.91,223.52 v44.45,223.52 v46.99,223.52
N$2011  (via drill 0.94)
  Bottom 2.032: v36.83,226.06 v39.37,226.06 v41.91,226.06 v44.45,226.06 v46.99,226.06
N$2012  (via drill 0.94)
  Bottom 2.032: v36.83,228.6 v39.37,228.6 v41.91,228.6 v44.45,228.6 v46.99,228.6
N$2013  (via drill 0.94)
  Bottom 2.032: v36.83,231.14 v39.37,231.14 v41.91,231.14 v44.45,231.14 v46.99,231.14
N$2014  (via drill 0.94)
  Bottom 2.032: v36.83,233.68 v39.37,233.68 v41.91,233.68 v44.45,233.68 v46.99,233.68
N$2015  (via drill 0.94)
  Bottom 2.032: v36.83,236.22 v39.37,236.22 v41.91,236.22 v44.45,236.22 v46.99,236.22
N$2016  (via drill 0.94)
  Bottom 2.032: v36.83,238.76 v39.37,238.76 v41.91,238.76 v44.45,238.76 v46.99,238.76
N$2017  (via drill 0.94)
  Bottom 2.032: v36.83,241.3 v39.37,241.3 v41.91,241.3 v44.45,241.3 v46.99,241.3
N$2018  (via drill 0.94)
  Bottom 2.032: v36.83,243.84 v39.37,243.84 v41.91,243.84 v44.45,243.84 v46.99,243.84
N$2019  (via drill 0.94)
  Bottom 2.032: v36.83,246.38 v39.37,246.38 v41.91,246.38 v44.45,246.38 v46.99,246.38
N$2020  (via drill 0.94)
  Bottom 2.032: v36.83,248.92 v39.37,248.92 v41.91,248.92 v44.45,248.92 v46.99,248.92
N$2021  (via drill 0.94)
  Bottom 2.032: v36.83,251.46 v39.37,251.46 v41.91,251.46 v44.45,251.46 v46.99,251.46
N$2022  (via drill 0.94)
  Bottom 2.032: v36.83,254 v39.37,254 v41.91,254 v44.45,254 v46.99,254
N$2023  (via drill 0.94)
  Bottom 2.032: v36.83,256.54 v39.37,256.54 v41.91,256.54 v44.45,256.54 v46.99,256.54
N$2024  (via drill 0.94)
  Bottom 2.032: v36.83,259.08 v39.37,259.08 v41.91,259.08 v44.45,259.08 v46.99,259.08
N$2025  (via drill 0.94)
  Bottom 2.032: v36.83,261.62 v39.37,261.62 v41.91,261.62 v44.45,261.62 v46.99,261.62
N$2026  (via drill 0.94)
  Bottom 2.032: v36.83,264.16 v39.37,264.16 v41.91,264.16 v44.45,264.16 v46.99,264.16
N$2027  (via drill 0.94)
  Bottom 2.032: v36.83,266.7 v39.37,266.7 v41.91,266.7 v44.45,266.7 v46.99,266.7
N$2028  (via drill 0.94)
  Bottom 2.032: v36.83,269.24 v39.37,269.24 v41.91,269.24 v44.45,269.24 v46.99,269.24
N$2029  (via drill 0.94)
  Bottom 2.032: v36.83,271.78 v39.37,271.78 v41.91,271.78 v44.45,271.78 v46.99,271.78
N$2030  (via drill 0.94)
  Bottom 2.032: v36.83,274.32 v39.37,274.32 v41.91,274.32 v44.45,274.32 v46.99,274.32
N$2031  (via drill 0.94)
  Bottom 2.032: v36.83,276.86 v39.37,276.86 v41.91,276.86 v44.45,276.86 v46.99,276.86
N$2032  (via drill 0.94)
  Bottom 2.032: v36.83,10.16 v39.37,10.16 v41.91,10.16 v44.45,10.16 v46.99,10.16
N$2033  (via drill 0.94)
  Bottom 2.032: v36.83,279.4 v39.37,279.4 v41.91,279.4 v44.45,279.4 v46.99,279.4
N$2034  (via drill 0.94)
  Bottom 2.032: v19.05,12.7 v21.59,12.7 v24.13,12.7 v26.67,12.7 v29.21,12.7
N$2035  (via drill 0.94)
  Bottom 2.032: v19.05,15.24 v21.59,15.24 v24.13,15.24 v26.67,15.24 v29.21,15.24
N$2036  (via drill 0.94)
  Bottom 2.032: v19.05,17.78 v21.59,17.78 v24.13,17.78 v26.67,17.78 v29.21,17.78
N$2037  (via drill 0.94)
  Bottom 2.032: v19.05,20.32 v21.59,20.32 v24.13,20.32 v26.67,20.32 v29.21,20.32
N$2038  (via drill 0.94)
  Bottom 2.032: v19.05,22.86 v21.59,22.86 v24.13,22.86 v26.67,22.86 v29.21,22.86
N$2039  (via drill 0.94)
  Bottom 2.032: v19.05,25.4 v21.59,25.4 v24.13,25.4 v26.67,25.4 v29.21,25.4
N$2040  (via drill 0.94)
  Bottom 2.032: v19.05,27.94 v21.59,27.94 v24.13,27.94 v26.67,27.94 v29.21,27.94
N$2041  (via drill 0.94)
  Bottom 2.032: v19.05,30.48 v21.59,30.48 v24.13,30.48 v26.67,30.48 v29.21,30.48
N$2042  (via drill 0.94)
  Bottom 2.032: v19.05,33.02 v21.59,33.02 v24.13,33.02 v26.67,33.02 v29.21,33.02
N$2043  (via drill 0.94)
  Bottom 2.032: v19.05,35.56 v21.59,35.56 v24.13,35.56 v26.67,35.56 v29.21,35.56
N$2044  (via drill 0.94)
  Bottom 2.032: v19.05,38.1 v21.59,38.1 v24.13,38.1 v26.67,38.1 v29.21,38.1
N$2045  (via drill 0.94)
  Bottom 2.032: v19.05,40.64 v21.59,40.64 v24.13,40.64 v26.67,40.64 v29.21,40.64
N$2046  (via drill 0.94)
  Bottom 2.032: v19.05,43.18 v21.59,43.18 v24.13,43.18 v26.67,43.18 v29.21,43.18
N$2047  (via drill 0.94)
  Bottom 2.032: v19.05,45.72 v21.59,45.72 v24.13,45.72 v26.67,45.72 v29.21,45.72
N$2048  (via drill 0.94)
  Bottom 2.032: v19.05,48.26 v21.59,48.26 v24.13,48.26 v26.67,48.26 v29.21,48.26
N$2049  (via drill 0.94)
  Bottom 2.032: v19.05,50.8 v21.59,50.8 v24.13,50.8 v26.67,50.8 v29.21,50.8
N$2050  (via drill 0.94)
  Bottom 2.032: v19.05,53.34 v21.59,53.34 v24.13,53.34 v26.67,53.34 v29.21,53.34
N$2051  (via drill 0.94)
  Bottom 2.032: v19.05,55.88 v21.59,55.88 v24.13,55.88 v26.67,55.88 v29.21,55.88
N$2052  (via drill 0.94)
  Bottom 2.032: v19.05,58.42 v21.59,58.42 v24.13,58.42 v26.67,58.42 v29.21,58.42
N$2053  (via drill 0.94)
  Bottom 2.032: v19.05,60.96 v21.59,60.96 v24.13,60.96 v26.67,60.96 v29.21,60.96
N$2054  (via drill 0.94)
  Bottom 2.032: v19.05,63.5 v21.59,63.5 v24.13,63.5 v26.67,63.5 v29.21,63.5
N$2055  (via drill 0.94)
  Bottom 2.032: v19.05,66.04 v21.59,66.04 v24.13,66.04 v26.67,66.04 v29.21,66.04
N$2056  (via drill 0.94)
  Bottom 2.032: v19.05,68.58 v21.59,68.58 v24.13,68.58 v26.67,68.58 v29.21,68.58
N$2057  (via drill 0.94)
  Bottom 2.032: v19.05,71.12 v21.59,71.12 v24.13,71.12 v26.67,71.12 v29.21,71.12
N$2058  (via drill 0.94)
  Bottom 2.032: v19.05,73.66 v21.59,73.66 v24.13,73.66 v26.67,73.66 v29.21,73.66
N$2059  (via drill 0.94)
  Bottom 2.032: v19.05,76.2 v21.59,76.2 v24.13,76.2 v26.67,76.2 v29.21,76.2
N$2060  (via drill 0.94)
  Bottom 2.032: v19.05,78.74 v21.59,78.74 v24.13,78.74 v26.67,78.74 v29.21,78.74
N$2061  (via drill 0.94)
  Bottom 2.032: v19.05,81.28 v21.59,81.28 v24.13,81.28 v26.67,81.28 v29.21,81.28
N$2062  (via drill 0.94)
  Bottom 2.032: v19.05,83.82 v21.59,83.82 v24.13,83.82 v26.67,83.82 v29.21,83.82
N$2063  (via drill 0.94)
  Bottom 2.032: v19.05,86.36 v21.59,86.36 v24.13,86.36 v26.67,86.36 v29.21,86.36
N$2064  (via drill 0.94)
  Bottom 2.032: v19.05,88.9 v21.59,88.9 v24.13,88.9 v26.67,88.9 v29.21,88.9
N$2065  (via drill 0.94)
  Bottom 2.032: v19.05,91.44 v21.59,91.44 v24.13,91.44 v26.67,91.44 v29.21,91.44
N$2066  (via drill 0.94)
  Bottom 2.032: v19.05,93.98 v21.59,93.98 v24.13,93.98 v26.67,93.98 v29.21,93.98
N$2067  (via drill 0.94)
  Bottom 2.032: v19.05,96.52 v21.59,96.52 v24.13,96.52 v26.67,96.52 v29.21,96.52
N$2068  (via drill 0.94)
  Bottom 2.032: v19.05,99.06 v21.59,99.06 v24.13,99.06 v26.67,99.06 v29.21,99.06
N$2069  (via drill 0.94)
